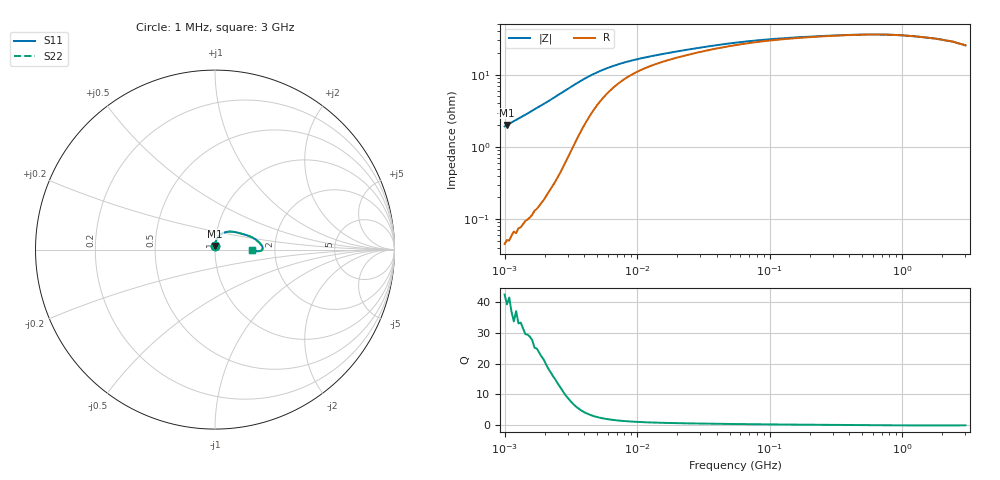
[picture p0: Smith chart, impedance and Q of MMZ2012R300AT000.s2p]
! S-parameter Generated by TDK Corporation
! Copyright(C) 2016 TDK Corporation.
! All Rights Reserved.
! TDK P/N: MMZ2012R300AT000 (Chip Beads)
! Property: |Z|=30¶ at 100MHz
! Size(LxWxT): 2x1.25x0.85mm, 0.079x0.049x0.033inches
! Model Type: s2p (Touchstone File Format Version 1.0)
! Frequency: DC=Yes Start=1MHz Stop=3000MHz 202points Log-sweep
! Note: This model was converted from impedance.
! Model Generated on May. 16, 2016
! Hash(MD5):
! Port Assignments:
!  1 ---@@@--- 2
! Applicable Conditions:
!  Temperature = 25 degC
!  DC Bias Current = 0 A
!  Small Signal Operation
! Terms and conditions regarding TDK Simulation Models
! (1)This simulation model is being provided solely for informational purposes. Please refer to the specifications of the products in terms of detailed characteristics of such products.
! (2)In no event shall TDK Corporation of any of its subsidiaries be liable for any loss or damage arising, directly or indirectly,
!  From any information contained in this simulation model, including, but not limited to loss or damages arising from any inaccuracies, omissions or errors in connection with such information.
! (3)Any and all copyrights on this simulation model are owned by TDK Corporation.
!  Duplication or redistribution of this simulation model without prior written permission from TDK Corporation is prohibited.
! (4)This simulation model is subject to any modification or change without any prior notice.
! (5)Neither TDK Corporation nor any of its subsidiaries shall make any warranty, express or implied,
!  Including but not limited to the correctness, implied warranties of merchantability and fitness for a particular purpose with respect to this simulation models.
! (6)The use of this simulation model shall be deemed to have consented to the terms and conditions hereof.
# MHz S MA R 50
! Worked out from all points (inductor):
!   201 points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, 1 MHz to 3 GHz, reference 50 ohm
!   read as one part in series: L = 309 nH near 1.041 MHz
!   highest Q = 41.5 at 1.041 MHz (marker M1), where L = 307 nH
!   self-resonance near 844.1 MHz
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1  0.01926 87.5  0.9994 -1.1  0.9994 -1.1  0.01926 87.5
1.040844  0.0201 87.4  0.9993 -1.2  0.9993 -1.2  0.0201 87.4
1.682724  0.03308 85.8  0.9981 -1.9  0.9981 -1.9  0.03308 85.8
2.511129  0.05153 82.9  0.9949 -2.9  0.9949 -2.9  0.05153 82.9
3.32329  0.07095 77.5  0.9871 -4.0  0.9871 -4.0  0.07095 77.5
3.900413  0.08385 72.8  0.9784 -4.7  0.9784 -4.7  0.08385 72.8
4.57776  0.09686 67.1  0.9664 -5.3  0.9664 -5.3  0.09686 67.1
5.161903  0.1062 62.6  0.9558 -5.7  0.9558 -5.7  0.1062 62.6
5.820586  0.115 58.2  0.9446 -5.9  0.9446 -5.9  0.115 58.2
6.83139  0.1256 52.7  0.9292 -6.2  0.9292 -6.2  0.1256 52.7
9.410094  0.1439 43.2  0.9005 -6.3  0.9005 -6.3  0.1439 43.2
14.61624  0.1647 33.8  0.868 -6.1  0.868 -6.1  0.1647 33.8
30.0453  0.1962 23.9  0.8244 -5.5  0.8244 -5.5  0.1962 23.9
54.77226  0.22 17.5  0.793 -4.8  0.793 -4.8  0.22 17.5
99.84923  0.2384 12.4  0.7689 -3.8  0.7689 -3.8  0.2384 12.4
213.6344  0.2543 7.5  0.7487 -2.5  0.7487 -2.5  0.2543 7.5
475.755  0.2646 3.3  0.736 -1.2  0.736 -1.2  0.2646 3.3
800.5644  0.264 0.3  0.736 -0.1  0.736 -0.1  0.264 0.3
1102.76  0.2578 -1.3  0.7423 0.4  0.7423 0.4  0.2578 -1.3
1782.824  0.2406 -2.1  0.7596 0.7  0.7596 0.7  0.2406 -2.1
2455.801  0.2224 -1.8  0.7778 0.5  0.7778 0.5  0.2224 -1.8
3000  0.2035 -0.0  0.7965 0.0  0.7965 0.0  0.2035 -0.0
